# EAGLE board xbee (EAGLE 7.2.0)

Size 25.4 x 27.94 mm. Coordinates in mm from the lower left corner, seen from the top.
Outline: 0,0 25.07,0
Outline: 0,21.58 0,0
Outline: 0,0 25.4,0 25.4,21.59 17.78,27.94 7.62,27.94 0,21.59 0,0
Copper layers (1*16): Top 0.035mm / dielectric 1.5mm / Bottom 0.035mm
Design rules "default": minimum track width 10mil, minimum drill 24mil, track to track 8mil, track to pad 8mil, pad to pad 8mil, via to via 8mil, smd to smd 8mil, copper to edge 40mil, drill to drill 8mil, minimum pad ring 10mil, minimum via ring 8mil, stop-mask expansion 4mil, vias tented up to drill 0mil, thermal gap 10mil

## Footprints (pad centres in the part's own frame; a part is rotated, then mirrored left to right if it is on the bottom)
XBEE-SILK = drill 0.8 pad 1.524: 1 -11,20; 2 -11,18; 3 -11,16; 4 -11,14; 5 -11,12; 6 -11,10; 7 -11,8; 8 -11,6; 9 -11,4; 10 -11,2; 11 11,2; 12 11,4; 13 11,6; 14 11,8; 15 11,10; 16 11,12; 17 11,14; 18 11,16; 19 11,18; 20 11,20
ESP-03 = smd 1 x 1.5: ANT 4,12.4; CH_PD 6,12.4; GND 16,12.4; GPIO0 16,-0.2; GPIO2 14,-0.2; GPIO12 8,-0.2; GPIO13 10,-0.2; GPIO14 6,-0.2; GPIO15 12,-0.2; GPIO18 8,12.4; NC 14,12.4; URXD 10,12.4; UTXD 12,12.4; VCC 4,-0.2

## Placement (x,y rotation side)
U$1  XBEE-1B2  [XBEE-SILK]  12.7,0 0 top
U$2  ESP8266  [ESP-03]  19.05,5.08 90 top

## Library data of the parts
U$1 = SparkFun-RF
U$2 = ESP8266

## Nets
GND: U$1.10
VDD: U$1.1

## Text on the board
Dimension: Safecast WiFi

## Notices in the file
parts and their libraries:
SparkFun-RF: Licensing: Creative Commons ShareAlike 4.0 International - https://creativecommons.org/licenses/by-sa/4.0
